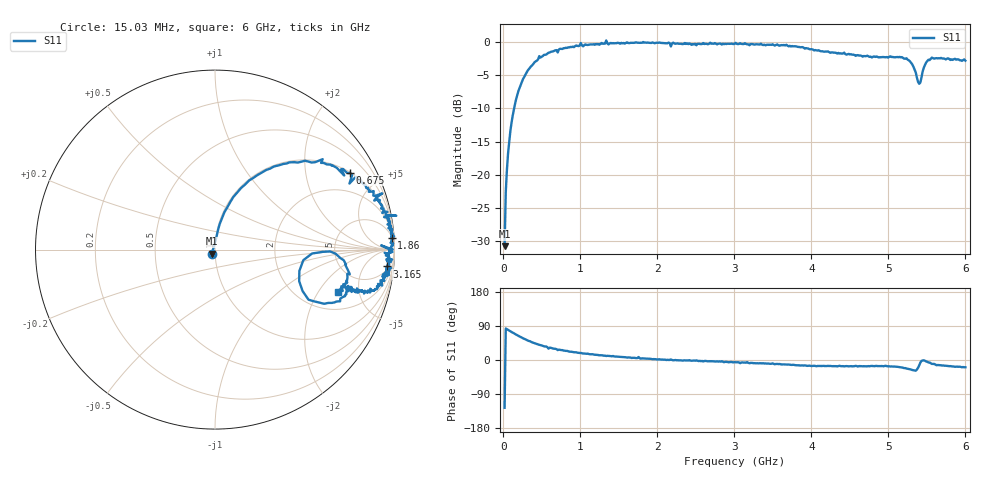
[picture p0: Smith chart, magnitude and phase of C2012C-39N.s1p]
!	Network	Analyzer	HP8753E.07.74:	Oct	30	2002	Serial	No.	JP38451487
!	Hewlett-Packard
!	7	Sep	2009	10:54:08
!	Frequency	S11
#	HZ	S	RI	R	50
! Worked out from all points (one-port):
!   400 points, 15.03 MHz to 6 GHz, reference 50 ohm
!   lowest |S11| = -30.7 dB at 15.03 MHz (marker M1), VSWR 1.06, Z = 48.3 - j2.27 ohm
!   |S11| at or under -10 dB: start of sweep to 138 MHz
!   S11 on the Smith chart (normalised r, x): 15.03 MHz: 0.97, -0.05; 675 MHz: 1.02, +3.50; 1.86 GHz: 6, +30; 3.165 GHz: 7, -18; 6 GHz: 3.05, -3.04
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1.502992e7  -0.0171 -0.0235
3.002985e7  0.00879 0.0734
6.00297e7  0.0263 0.143
1.050295e8  0.0694 0.237
1.650292e8  0.145 0.343
3.450283e8  0.415 0.486
4.650277e8  0.6 0.504
6.750266e8  0.753 0.429
7.650262e8  0.796 0.39
1.335023e9  1.01 0.189
1.365023e9  0.942 0.181
1.515022e9  0.961 0.14
1.860021e9  0.985 0.0629
2.175019e9  0.926 0.0235
2.265019e9  0.976 -0.00958
3.015015e9  0.981 -0.103
3.165014e9  0.957 -0.094
3.765011e9  0.906 -0.202
4.515007e9  0.777 -0.226
4.965005e9  0.741 -0.202
5.265004e9  0.666 -0.294
5.355003e9  0.521 -0.279
5.385003e9  0.469 -0.176
5.430003e9  0.541 -0.0217
5.460003e9  0.641 -0.0101
5.520002e9  0.73 -0.0831
5.625002e9  0.734 -0.182
6e9  0.684 -0.237
